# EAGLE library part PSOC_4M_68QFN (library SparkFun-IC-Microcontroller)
PSoC 4200 CY8C4247LTI PSoC4200M Datasheet SparkFun Products Spectacle Directory Board () ProSoC Mini () Prototype in process! Do keep!
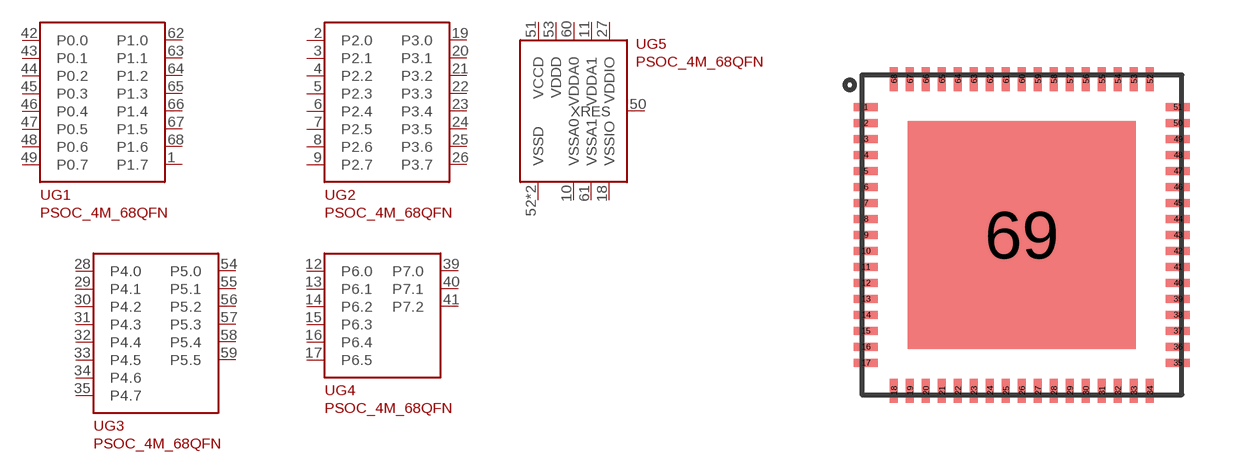
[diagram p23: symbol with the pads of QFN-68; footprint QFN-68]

Designator prefix U; gates G1=CY8C42M-68QFN_P0_P1 G2=CY8C42M-68QFN_P2_P3 G3=CY8C42M-68QFN_P4_P5 G4=CY8C42M-68QFN_P6_P7 G5=CY8C42M-68QFN_POWER

## PSOC_4M_68QFN (PROD_ID: IC-13259; VALUE: CY8C4247LTI)  [QFN-68]
1  G1:P1.7
2  G2:P2.0
3  G2:P2.1
4  G2:P2.2
5  G2:P2.3
6  G2:P2.4
7  G2:P2.5
8  G2:P2.6
9  G2:P2.7
10  G5:VSSA0
11  G5:VDDA1
12  G4:P6.0
13  G4:P6.1
14  G4:P6.2
15  G4:P6.3
16  G4:P6.4
17  G4:P6.5
18  G5:VSSIO
19  G2:P3.0
20  G2:P3.1
21  G2:P3.2
22  G2:P3.3
23  G2:P3.4
24  G2:P3.5
25  G2:P3.6
26  G2:P3.7
27  G5:VDDIO
28  G3:P4.0
29  G3:P4.1
30  G3:P4.2
31  G3:P4.3
32  G3:P4.4
33  G3:P4.5
34  G3:P4.6
35  G3:P4.7
39  G4:P7.0
40  G4:P7.1
41  G4:P7.2
42  G1:P0.0
43  G1:P0.1
44  G1:P0.2
45  G1:P0.3
46  G1:P0.4
47  G1:P0.5
48  G1:P0.6
49  G1:P0.7
50  G5:XRES
51  G5:VCCD
52  G5:VSSD
53  G5:VDDD
54  G3:P5.0
55  G3:P5.1
56  G3:P5.2
57  G3:P5.3
58  G3:P5.4
59  G3:P5.5
60  G5:VDDA0
61  G5:VSSA1
62  G1:P1.0
63  G1:P1.1
64  G1:P1.2
65  G1:P1.3
66  G1:P1.4
67  G1:P1.5
68  G1:P1.6
69  G5:VSSD

## Footprint QFN-68 (pad centres in mm)
smd 0.6 x 0.2: 1 -3.9,3.2; 2 -3.9,2.8; 3 -3.9,2.4; 4 -3.9,2; 5 -3.9,1.6; 6 -3.9,1.2; 7 -3.9,0.8; 8 -3.9,0.4; 9 -3.9,0; 10 -3.9,-0.4; 11 -3.9,-0.8; 12 -3.9,-1.2; 13 -3.9,-1.6; 14 -3.9,-2; 15 -3.9,-2.4; 16 -3.9,-2.8; 17 -3.9,-3.2; 35 3.9,-3.2; 36 3.9,-2.8; 37 3.9,-2.4; 38 3.9,-2; 39 3.9,-1.6; 40 3.9,-1.2; 41 3.9,-0.8; 42 3.9,-0.4; 43 3.9,0; 44 3.9,0.4; 45 3.9,0.8; 46 3.9,1.2; 47 3.9,1.6; 48 3.9,2; 49 3.9,2.4; 50 3.9,2.8; 51 3.9,3.2
smd 0.2 x 0.6: 18 -3.2,-3.9; 19 -2.8,-3.9; 20 -2.4,-3.9; 21 -2,-3.9; 22 -1.6,-3.9; 23 -1.2,-3.9; 24 -0.8,-3.9; 25 -0.4,-3.9; 26 0,-3.9; 27 0.4,-3.9; 28 0.8,-3.9; 29 1.2,-3.9; 30 1.6,-3.9; 31 2,-3.9; 32 2.4,-3.9; 33 2.8,-3.9; 34 3.2,-3.9; 52 3.2,3.9; 53 2.8,3.9; 54 2.4,3.9; 55 2,3.9; 56 1.6,3.9; 57 1.2,3.9; 58 0.8,3.9; 59 0.4,3.9; 60 0,3.9; 61 -0.4,3.9; 62 -0.8,3.9; 63 -1.2,3.9; 64 -1.6,3.9; 65 -2,3.9; 66 -2.4,3.9; 67 -2.8,3.9; 68 -3.2,3.9
smd 5.7 x 5.7: 69 0,0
